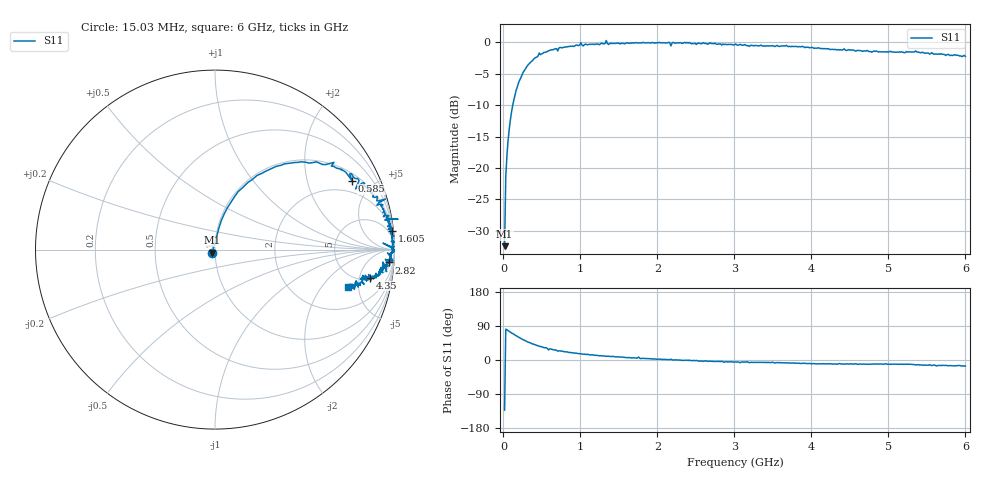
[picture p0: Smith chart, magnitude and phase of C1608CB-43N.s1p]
!	Network	Analyzer	HP8753E.07.74:	Oct	30	2002	Serial	No.	JP38451487
!	Hewlett-Packard
!	28	Aug	2009	8:10:37
!	Frequency	S11
#	HZ	S	RI	R	50
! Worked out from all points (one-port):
!   400 points, 15.03 MHz to 6 GHz, reference 50 ohm
!   lowest |S11| = -32.4 dB at 15.03 MHz (marker M1), VSWR 1.05, Z = 48.4 - j1.71 ohm
!   |S11| at or under -10 dB: start of sweep to 120.8 MHz
!   S11 on the Smith chart (normalised r, x): 15.03 MHz: 0.97, -0.03; 585 MHz: 1.34, +3.80; 1.605 GHz: 1, +19; 2.82 GHz: 9, -23; 4.35 GHz: 5.36, -7.19; 6 GHz: 3.67, -3.81
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1.502992e7  -0.0161 -0.0177
3.002985e7  0.0126 0.0842
4.502978e7  0.0226 0.123
9.002955e7  0.0682 0.232
1.350293e8  0.129 0.323
2.10029e8  0.261 0.425
3.450283e8  0.478 0.489
5.550272e8  0.705 0.447
5.850271e8  0.765 0.382
7.650262e8  0.828 0.36
1.005025e9  0.951 0.282
1.320023e9  0.96 0.175
1.335023e9  1.02 0.169
1.365023e9  0.946 0.165
1.515022e9  0.961 0.129
1.605022e9  0.988 0.103
1.755021e9  0.977 0.136
1.785021e9  0.986 0.0631
2.145019e9  0.999 0.0177
2.175019e9  0.936 0.0359
2.265019e9  0.992 0.00101
2.820016e9  0.968 -0.0713
3.015015e9  0.965 -0.0911
3.765011e9  0.916 -0.125
4.350008e9  0.862 -0.156
4.515007e9  0.858 -0.152
5.265004e9  0.822 -0.163
6e9  0.743 -0.21
